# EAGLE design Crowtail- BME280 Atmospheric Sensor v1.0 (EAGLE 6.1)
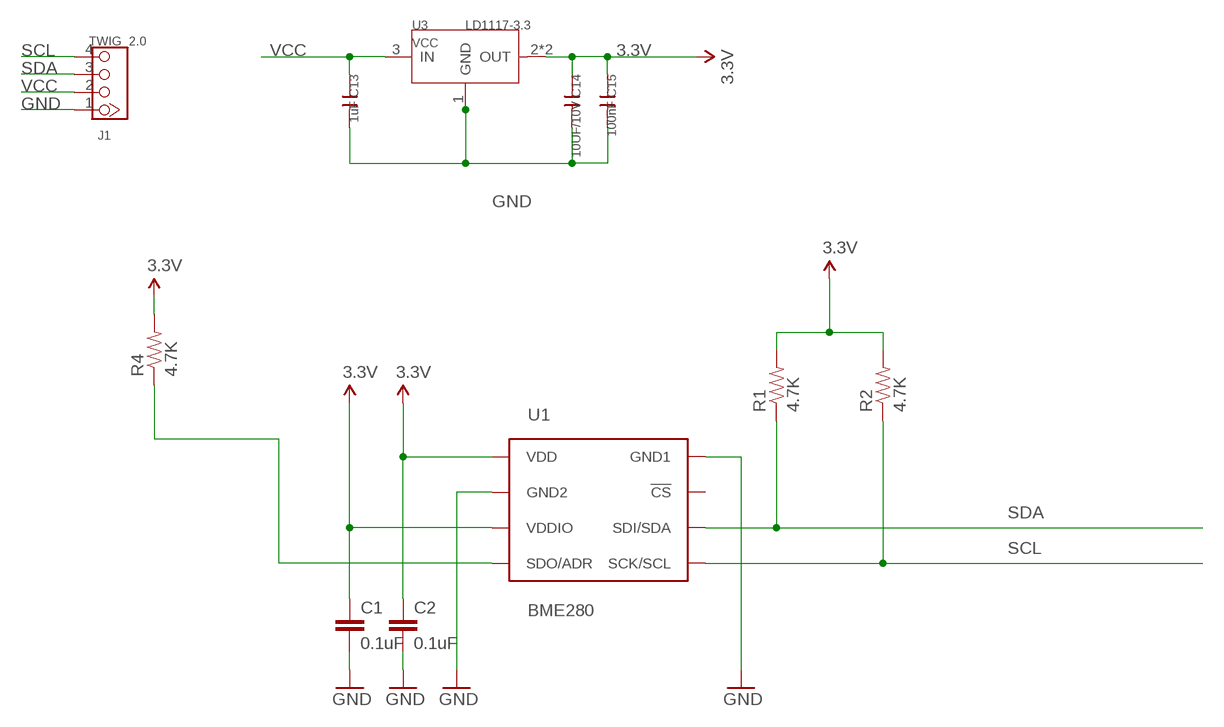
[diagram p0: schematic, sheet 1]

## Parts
C1  0.1uF  0.1UF-25V-5%(0603)  [0603-CAP]
C2  0.1uF  0.1UF-25V-5%(0603)  [0603-CAP]
C13  1uF  C-0603  [C0603]
C14  10UF/10V  C-0805  [C0805]
C15  100nF  C-0603  [C0603]
J1  TWIG_2.0  [2.0_1X4]
R1  4.7K  4.7KOHM-1/10W-1%(0603)  [0603-RES]
R2  4.7K  4.7KOHM-1/10W-1%(0603)  [0603-RES]
R4  4.7K  4.7KOHM-1/10W-1%(0603)  [0603-RES]
U1  BME280  [BME280_LGA]
U3  LD1117-3.3  LD1117'SOT89'  [SOT89]

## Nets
3.3V: C1.1 C2.1 C14.1 C15.1 R1.2 R2.2 R4.2 U1.P$6(VDDIO) U1.P$8(VDD) U3.2(OUT) U3.4(OUT)
GND: C1.2 C2.2 C13.2 C14.2 C15.2 J1.1 U1.P$1(GND1) U1.P$7(GND2) U3.1(GND)
SCL: J1.4 R2.1 U1.P$4(SCK/SCL)
SDA: J1.3 R1.1 U1.P$3(SDI/SDA)
SDO/ADR: R4.1 U1.P$5(SDO/ADR)
VCC: C13.1 J1.2 U3.3(IN)
Unconnected: U1.P$2(!CS)

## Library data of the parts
C1 C2 = SparkFun-Capacitors:0.1UF-25V-5%(0603): CAP-08604; PROD_ID: CAP-08604
C13-C15 = Discrete:C*: Ceramic Capacitors
J1 = CONNECTER:TWIG_2.0
R1 R2 R4 = SparkFun-Resistors:4.7KOHM-1/10W-1%(0603): RES-07857; PROD_ID: RES-07857
U1 = BME280ComponentLibrary:BME280; PROD_ID: IC-13090
U3 = IC:LD1117: Low Drop Fixed And Adjustable Positive Voltage Regulators http://www.datasheetcatalog.org/datasheet/SGSThomsonMicroelectronics/mXuqtqv.pdf

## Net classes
0 default: width 0.203 mm, drill 0.305 mm, clearance 0.203 mm
3 usbvcc: width 0.203 mm, drill 0.305 mm, clearance 0.203 mm

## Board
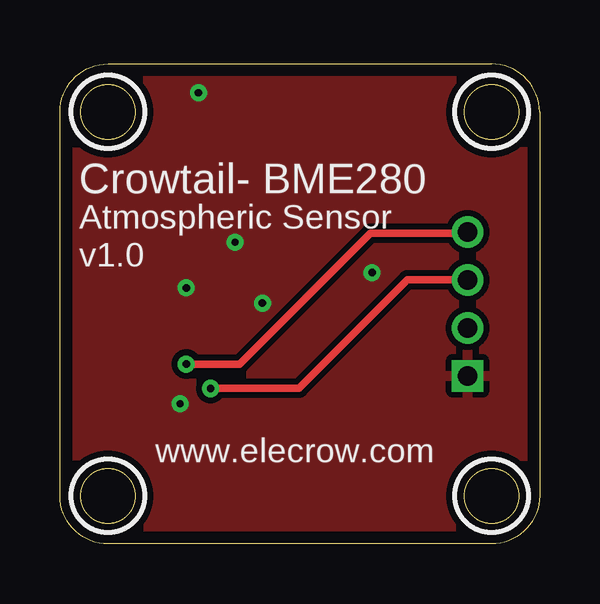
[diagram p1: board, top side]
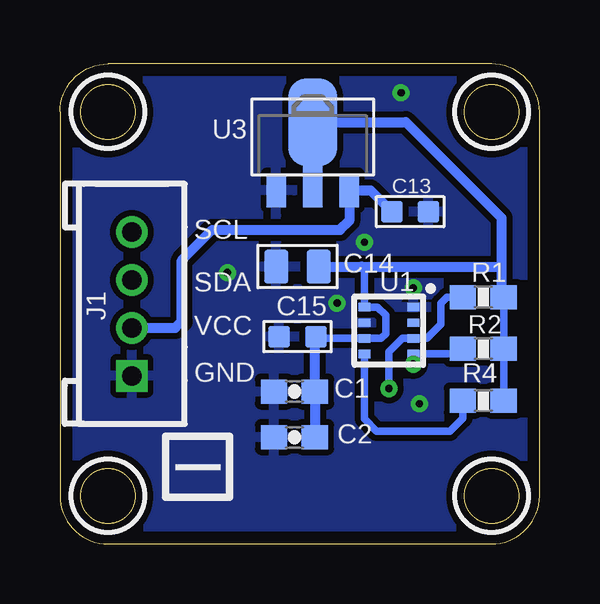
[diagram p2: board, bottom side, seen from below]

Size 20 x 20 mm. Coordinates in mm from the lower left corner, seen from the top.
Outline: 20,18 20,2 arc-90 18,0 2,0 arc-90 0,2 0,18 arc-90 2,20 18,20 arc-90 20,18
Outline: circle at 18,18 radius 1.14
Outline: circle at 18,2 radius 1.14
Outline: circle at 2,18 radius 1.14
Outline: circle at 2,2 radius 1.14
Copper layers (1*16): Top 0.035mm / dielectric 1.5mm / Bottom 0.035mm
Design rules: minimum track width 10mil, minimum drill 16mil, track to track 8mil, track to pad 8mil, pad to pad 8mil, via to via 8mil, smd to smd 8mil, copper to edge 20mil, drill to drill 8mil, minimum pad ring 10mil, minimum via ring 8mil, stop-mask expansion 4mil, vias tented up to drill 100mil, thermal gap 10mil
tRestrict: area 16.5,16.5 to 19.5,19.5; area 16.5,0.5 to 19.5,3.5; area 0.5,16.5 to 3.5,19.5; area 0.5,0.5 to 3.5,3.5
bRestrict: area 16.5,16.5 to 19.5,19.5; area 16.5,0.5 to 19.5,3.5; area 0.5,16.5 to 3.5,19.5; area 0.5,0.5 to 3.5,3.5

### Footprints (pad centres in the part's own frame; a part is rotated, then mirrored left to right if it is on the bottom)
0603-CAP = smd 1.1 x 1: 1 -0.85,0; 2 0.85,0
C0603 = smd 0.889 x 0.889: 1 -0.762,0; 2 0.762,0
C0805 = smd 1.016 x 1.397: 1 -0.889,0; 2 0.889,0
2.0_1X4 = drill 0.8 pad 1.27 square: 1 -3,0 | drill 0.8 pad 1.27: 2 -1,0; 3 1,0; 4 3,0
0603-RES = smd 1.1 x 1: 1 -0.85,0; 2 0.85,0
BME280_LGA = smd 0.5 x 0.35: P$1 1.025,0.975; P$2 1.025,0.325; P$3 1.025,-0.325; P$4 1.025,-0.975; P$5 -1.025,-0.975; P$6 -1.025,-0.325; P$7 -1.025,0.325; P$8 -1.025,0.975
SOT89 = smd 0.8 x 1.4: 1 -1.524,-1.905; 3 1.524,-1.905 | smd 0.8 x 1.9: 2 0,-1.651 | smd 2.032 x 3.65: 4 0,0.94

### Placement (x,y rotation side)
C1  10.22,6.35 180 bottom
C2  10.22,4.45 180 bottom
C13  5.39,13.84 0 bottom
C14  10.09,11.56 180 bottom
C15  10.09,8.64 180 bottom
J1  17,10 90 bottom
R1  2.35,10.29 0 bottom
R2  2.35,8.13 0 bottom
R4  2.35,5.97 0 bottom
U1  6.28,8.89 0 bottom
U3  9.46,16.64 0 bottom

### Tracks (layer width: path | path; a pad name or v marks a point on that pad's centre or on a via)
3.3V
  Bottom 0.305: 7.43,11.56 7.31,11.44 U1.P$8 6.75,9.87 6.41,9.53 6.41,8.76 6.61,8.56 U1.P$6 9.26,8.56 C15.1 | R4.2 R2.2 R1.2
  Bottom 0.406: 1.58,11.68 1.58,13.59 5.57,17.58 U3.4 U3.2 | 1.58,11.68 1.58,10.38 R1.2 | C14.1 7.43,11.56 1.71,11.56 1.58,11.68 | C15.1 9.37,8.6 C1.1 C2.1
GND  (via drill 0.3)
  other vias: 8.44,10.03 5.27,10.67 7.3,12.57 5.78,18.8 5.01,5.84 13.02,11.3
  pour Top (isolate 0.254): 20.51,-0.76 -0.45,-0.89 -0.32,20.32 20.64,20.45
  pour Bottom (isolate 0.254): 20.51,-0.89 -0.45,-0.89 -0.32,20.45 20.64,20.45
SCL  (via drill 0.3)
  Top 0.305: J1.4 16.95,12.95 12.95,12.95 7.49,7.49 v5.27,7.49
  Bottom 0.305: R2.1 3.41,7.92 U1.P$4 5.26,7.5 v5.27,7.49
SDA  (via drill 0.3)
  Top 0.305: v6.28,6.48 9.97,6.48 14.49,11 J1.3
  Bottom 0.305: R1.1 3.87,10.29 4.12,10.03 4.12,9.14 4.7,8.56 U1.P$3 5.72,8.56 6.28,8 v6.28,6.48
SDO/ADR
  Bottom 0.305: U1.P$5 7.31,5.22 6.79,4.7 3.74,4.7 3.2,5.25 R4.1
VCC
  Bottom 0.406: J1.2 15.19,9 14.92,9.27 14.92,11.81 13.65,13.08 8.32,13.08 7.93,13.46 U3.3 7.05,14.73 C13.1

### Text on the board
tPlace: Crowtail- BME280 | Atmospheric Sensor | v1.0 | www.elecrow.com
bPlace: SCL | SDA | VCC | GND | I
